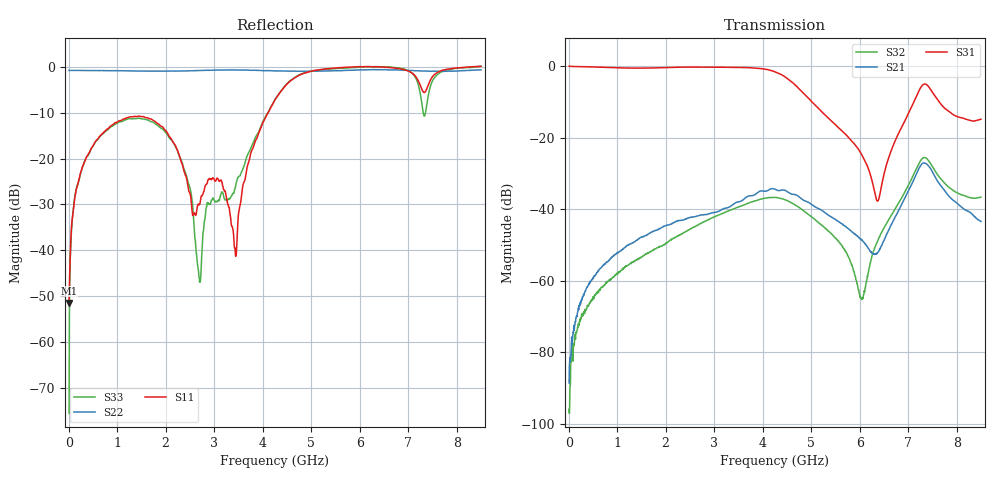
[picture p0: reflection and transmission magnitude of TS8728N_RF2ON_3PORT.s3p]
!Created with skrf (http://scikit-rf.org).
# GHz S RI R 50.0
!freq ReS11 ImS11 ReS12 ImS12 ReS13 ImS13
! ReS21 ImS21 ReS22 ImS22 ReS23 ImS23
! ReS31 ImS31 ReS32 ImS32 ReS33 ImS33
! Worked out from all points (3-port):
!   1601 points, 10 MHz to 8.5 GHz, reference 50 ohm
!   strongest paths, dB at 10 MHz, 2.132 GHz, 4.255 GHz, 6.378 GHz, 8.5 GHz:
!     S31: 0.0, -0.4, -1.6, -37.7, -14.9
!     S21: -88.7, -44.1, -34.5, -52.0, -43.5
!     S32: -96.0, -48.4, -36.8, -48.8, -36.7
!   lowest |S11| = -51.5 dB at 10 MHz (marker M1), VSWR 1.01, Z = 50.3 - j0.0139 ohm
!   |S11| at or under -10 dB: start of sweep to 4.112 GHz
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0.01  0.00265 -0.000138  1.61e-05 2.55e-05  0.9946 -0.00935
      1.95e-05 3.13e-05  -0.9169 0.00521  8.11e-06 1.88e-05
      0.9945 -0.00949  -1.46e-05 6.15e-06  0.000118 0.000116
0.1267375  0.00233 -0.0371  5.6e-06 0.000247  0.9808 -0.0649
           1.93e-05 0.000237  -0.9153 0.0433  5.89e-05 -0.000166
           0.9806 -0.0649  8.95e-06 -0.000167  0.0026 -0.0382
0.64675  -0.0606 -0.1656  -0.000208 0.00145  0.9158 -0.2947
         -0.000236 0.00145  -0.8924 0.1962  -0.000566 -0.000533
         0.9158 -0.2946  -0.000523 -0.000509  -0.0419 -0.169
2.137806  -0.0977 -0.122  4.2e-06 0.00629  0.5402 -0.7899
          1.85e-05 0.00626  -0.7067 0.5622  -0.00364 0.00117
          0.5405 -0.79  -0.00364 0.00116  -0.1305 -0.0845
2.694962  0.0295 -0.0113  0.00127 0.00808  0.2726 -0.9251
          0.00129 0.00806  -0.5781 0.709  -0.00488 0.00371
          0.2723 -0.9249  -0.00487 0.00373  0.00173 -0.00459
3.437838  -0.00213 -0.00879  0.00235 0.012  -0.197 -0.9367
          0.00233 0.0119  -0.4788 0.7943  -0.00348 0.00964
          -0.1974 -0.9363  -0.0035 0.00962  -0.00239 0.0487
4.255  -0.1986 0.391  0.0147 0.0119  -0.7199 -0.414
       0.0147 0.0119  -0.2688 0.8661  0.00839 0.0119
       -0.7198 -0.4126  0.00835 0.0119  -0.1502 0.4166
6.366887  0.3266 0.9512  0.000649 0.00233  -0.00624 -0.0113
          0.000644 0.00235  0.2657 0.8946  -0.00272 0.00226
          -0.00627 -0.0113  -0.00272 0.00224  0.3982 0.9271
7.306094  0.1774 0.511  0.0177 0.0401  -0.0638 -0.5439
          0.0178 0.0401  0.5087 0.7474  0.0203 0.0476
          -0.0651 -0.544  0.0202 0.0476  0.1749 0.2785
8.5  -0.3447 0.9565  0.00656 0.00146  -0.171 -0.0577
     0.00655 0.00148  0.7021 0.6101  0.0138 -0.00482
     -0.1706 -0.0575  0.0138 -0.00488  -0.3715 0.9504
